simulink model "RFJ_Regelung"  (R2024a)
settings: Solver=ode45  StartTime=0.0  StopTime=15  RelTol=1e-5  EnableMultiTasking=on
undefined symbols (not defined in the file or in its folder): sigbuilder_block

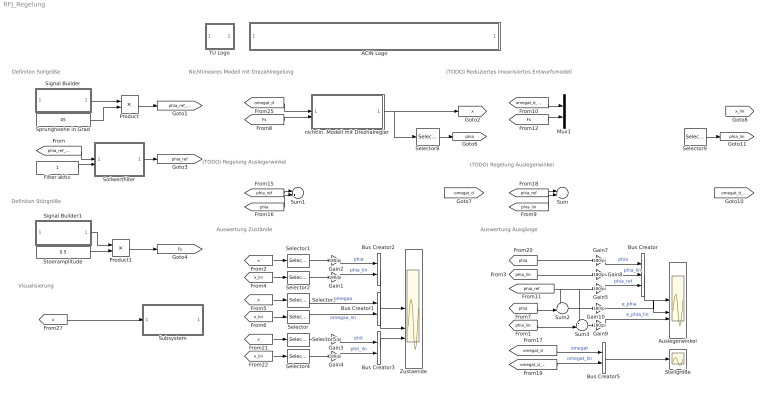
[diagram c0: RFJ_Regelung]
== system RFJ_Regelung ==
  note: Definiton Sollgröße
  note: Definiton Störgröße
  note: Nichtlineares Modell mit Drezahlregelung
  note: (TODO) Reduziertes linearisiertes Entwurfsmodell
  note: (TODO) Regelung Auslegerwinkel
  note: Auswertung Zustände
  note: Auswertung Ausgänge
  note: Visualisierung
  note: (TODO) Regelung Auslegerwinkel
  ACIN Logo : Subsystem
      mask init:
      | s = get_param(gcb,'UserData');
  Auslegerwinkel : Scope  NumInputPorts=3
  Bus Creator : BusCreator  Inputs=3
  Bus Creator{1..3,5} (4 alike) : BusCreator  Inputs=2
  Filter aktiv : Constant
  Gain{1..5,7..10} (9 alike) : Gain  Gain=180/pi
  Mux1 : Mux  Inputs=2
  Product : Product
  Product1 : Product
  Selector : Selector  InputPortWidth=3  IndexOptions=Index vector (dialog)  Indices=2  OutputSizes=1
  Selector1 : Selector  InputPortWidth=4  IndexOptions=Index vector (dialog)  Indices=1  OutputSizes=1
  Selector2 : Selector  InputPortWidth=3  IndexOptions=Index vector (dialog)  Indices=1  OutputSizes=1
  Selector3 : Selector  InputPortWidth=4  IndexOptions=Index vector (dialog)  Indices=2  OutputSizes=1
  Selector4 : Selector  InputPortWidth=3  IndexOptions=Index vector (dialog)  Indices=3  OutputSizes=1
  Selector5 : Selector  InputPortWidth=4  IndexOptions=Index vector (dialog)  Indices=3  OutputSizes=1
  Selector8 : Selector  InputPortWidth=4  IndexOptions=Index vector (dialog)  Indices=1  OutputSizes=1
  Selector9 : Selector  InputPortWidth=3  IndexOptions=Index vector (dialog)  Indices=1  OutputSizes=1
  Signal Builder : Subsystem  Tag=STV Subsys  LoadFcn=sigbuilder_block('load');  StartFcn=sigbuilder_block('start');  StopFcn=sigbuilder_block('stop');  ClipboardFcn=sigbuilder_block('clipboard');  mask(Sigbuilder block){tuvar=[0:10]}
      mask help: Simulink:masks:SigbuilderBlock_MD
      mask init:
      | if ~strcmp(get_param(bdroot(gcbh),'SimulationStatus'),'stopped') tuvar = sigbuilder_block('maskInit'); end
  Signal Builder1 : Subsystem  Tag=STV Subsys  LoadFcn=sigbuilder_block('load');  StartFcn=sigbuilder_block('start');  StopFcn=sigbuilder_block('stop');  ClipboardFcn=sigbuilder_block('clipboard');  mask(Sigbuilder block){tuvar=[0:10]}
      mask help: Simulink:masks:SigbuilderBlock_MD
      mask init:
      | if ~strcmp(get_param(bdroot(gcbh),'SimulationStatus'),'stopped') tuvar = sigbuilder_block('maskInit'); end
  Sollwertfilter : Subsystem
  Sprunghoehe in Grad : Constant  Value=45
  Stellgröße : Scope
  Stoeramplitude : Constant  Value=0.5
  Subsystem : Subsystem
  Sum : Sum  Inputs=|+-
  Sum1 : Sum  Inputs=|+-
  Sum2 : Sum  Inputs=-+|
  Sum3 : Sum  Inputs=-+|
  TU Logo : Subsystem
      mask init:
      | s = get_param(gcb,'UserData');
  Zustaende : Scope  NumInputPorts=3
  nichtlin. Modell mit Drezhalregler : Subsystem
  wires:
  Sum/1 -> ?
  [Fs] -> Mux1/2
  [omegat_d_lin] -> Mux1/1
  [Fs] -> nichtlin. Modell mit Drezhalregler/2(Fs)
  nichtlin. Modell mit Drezhalregler/1(x_red) -> Selector8/1, [x]
  ? -> Selector9/1, [x_lin]
  Mux1/1 -> ?
  Sum1/1 -> ?
  Sprunghoehe in Grad/1 -> Product/2
  Signal Builder/1(Signal 1) -> Product/1
  Product/1 -> [phia_ref_grad]
  [phia_ref_grad] -> Sollwertfilter/1(phia_ref_grad)
  Bus Creator1/1 -> Zustaende/2
  [x_lin] -> Selector/1
  [omegat_d] -> Bus Creator5/1  "omegat"
  [phia_lin] -> Gain8/1
  Selector/1 -> Bus Creator1/2  "omegaa_lin"
  Bus Creator5/1 -> Stellgröße/1
  Selector3/1 -> Bus Creator1/1  "omegaa"
  [omegat_d_lin] -> Bus Creator5/2  "omegat_lin"
  Bus Creator/1 -> Auslegerwinkel/1
  Selector1/1 -> Gain2/1
  [x_lin] -> Selector2/1
  Selector2/1 -> Gain1/1
  Selector5/1 -> Gain3/1
  Selector4/1 -> Gain4/1
  [x_lin] -> Selector4/1
  Bus Creator3/1 -> Zustaende/3
  Bus Creator2/1 -> Zustaende/1
  Gain2/1 -> Bus Creator2/1  "phia"
  Gain1/1 -> Bus Creator2/2  "phia_lin"
  Gain3/1 -> Bus Creator3/1  "phit"
  Gain4/1 -> Bus Creator3/2  "phit_lin"
  Gain5/1 -> Bus Creator/3  "phia_ref"
  Gain7/1 -> Bus Creator/1  "phia"
  Gain8/1 -> Bus Creator/2  "phia_lin"
  Gain10/1 -> Auslegerwinkel/2  "e_phia"
  Gain9/1 -> Auslegerwinkel/3  "e_phia_lin"
  Product1/1 -> [Fs]
  Signal Builder1/1(Signal 1) -> Product1/1
  Stoeramplitude/1 -> Product1/2
  Selector8/1 -> [phia]
  Selector9/1 -> [phia_lin]
  [omegat_d] -> nichtlin. Modell mit Drezhalregler/1(omegat)
  [phia_ref] -> Sum1/1
  [phia] -> Sum1/2
  [phia_ref] -> Sum/1
  [phia_lin] -> Sum/2
  Sum3/1 -> Gain9/1
  [phia_lin] -> Sum3/2
  [phia_ref] -> Sum2/1, Sum3/1, Gain5/1
  Sum2/1 -> Gain10/1
  Sollwertfilter/1(phia_ref) -> [phia_ref]
  ? -> [omegat_d]
  ? -> [omegat_d_lin]
  [phia] -> Sum2/2
  [phia] -> Gain7/1
  [x] -> Selector3/1
  [x] -> Selector1/1
  [x] -> Selector5/1
  [x] -> Subsystem/1(x)
  Filter aktiv/1 -> Sollwertfilter/2(act)

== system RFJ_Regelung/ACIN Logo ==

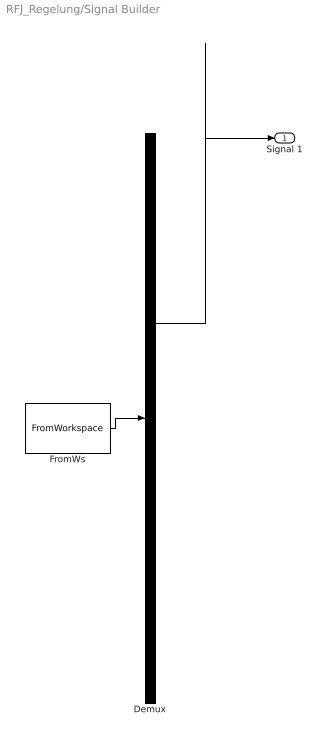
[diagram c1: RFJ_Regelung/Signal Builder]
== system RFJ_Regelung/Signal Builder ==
  Demux : Demux  Tag=STV Demux  Outputs=1
  FromWs : FromWorkspace  Tag=STV FromWs  VariableName=tuvar
  Signal 1 : Outport  Tag=STV Outport
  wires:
  Demux/1 -> Signal 1/1
  FromWs/1 -> Demux/1

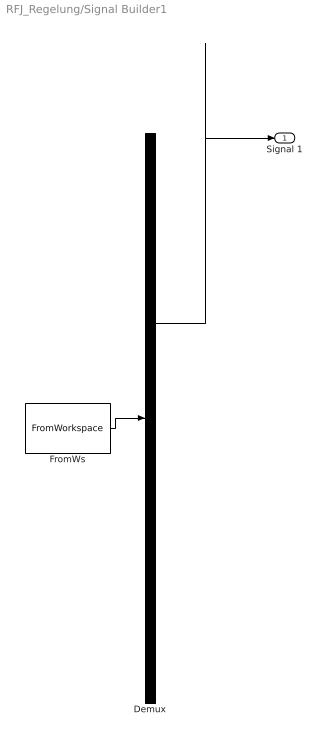
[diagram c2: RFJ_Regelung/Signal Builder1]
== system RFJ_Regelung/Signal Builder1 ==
  Demux : Demux  Tag=STV Demux  Outputs=1
  FromWs : FromWorkspace  Tag=STV FromWs  VariableName=tuvar
  Signal 1 : Outport  Tag=STV Outport
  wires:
  FromWs/1 -> Demux/1
  Demux/1 -> Signal 1/1

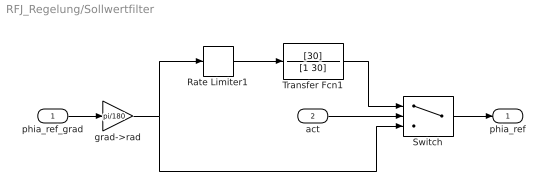
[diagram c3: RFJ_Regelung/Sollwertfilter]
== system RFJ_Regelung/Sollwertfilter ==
  phia_ref_grad : Inport
  act : Inport  Port=2
  Rate Limiter1 : RateLimiter  RisingSlewLimit=15  FallingSlewLimit=-15  SampleTimeMode=inherited
  Switch : Switch  Criteria=u2 > Threshold
  Transfer Fcn1 : TransferFcn  Numerator=[30]  Denominator=[1 30]
  grad->rad : Gain  Gain=pi/180
  phia_ref : Outport
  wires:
  phia_ref_grad/1 -> grad->rad/1
  grad->rad/1 -> Switch/3, Rate Limiter1/1
  Switch/1 -> phia_ref/1
  act/1 -> Switch/2
  Rate Limiter1/1 -> Transfer Fcn1/1
  Transfer Fcn1/1 -> Switch/1

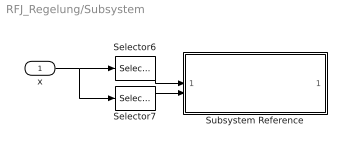
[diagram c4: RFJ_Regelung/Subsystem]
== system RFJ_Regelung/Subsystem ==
  x : Inport
  Selector6 : Selector  InputPortWidth=4  IndexOptions=Index vector (dialog)  Indices=1  OutputSizes=1
  Selector7 : Selector  InputPortWidth=4  IndexOptions=Index vector (dialog)  Indices=3  OutputSizes=1
  Subsystem Reference : Subsystem  ReferencedSubsystem=Visualisierung
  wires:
  Selector7/1 -> Subsystem Reference/2
  x/1 -> Selector7/1, Selector6/1
  Selector6/1 -> Subsystem Reference/1

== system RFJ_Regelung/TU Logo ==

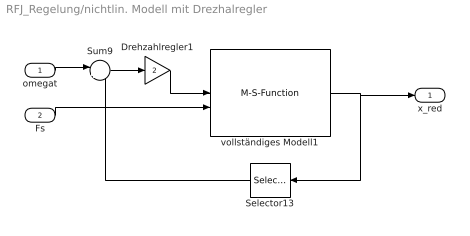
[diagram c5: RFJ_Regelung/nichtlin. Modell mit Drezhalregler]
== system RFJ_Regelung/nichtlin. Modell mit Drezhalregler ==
  omegat : Inport
  Fs : Inport  Port=2
  Drehzahlregler1 : Gain  Gain=2
  Selector13 : Selector  InputPortWidth=4  IndexOptions=Index vector (dialog)  Indices=4  OutputSizes=1
  Sum9 : Sum  Inputs=|+-
  vollständiges Modell1 : M-S-Function  FunctionName=RFJ_Student_S
  x_red : Outport
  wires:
  Selector13/1 -> Sum9/2
  Drehzahlregler1/1 -> vollständiges Modell1/1
  Fs/1 -> vollständiges Modell1/2
  Sum9/1 -> Drehzahlregler1/1
  omegat/1 -> Sum9/1
  vollständiges Modell1/1 -> Selector13/1, x_red/1
